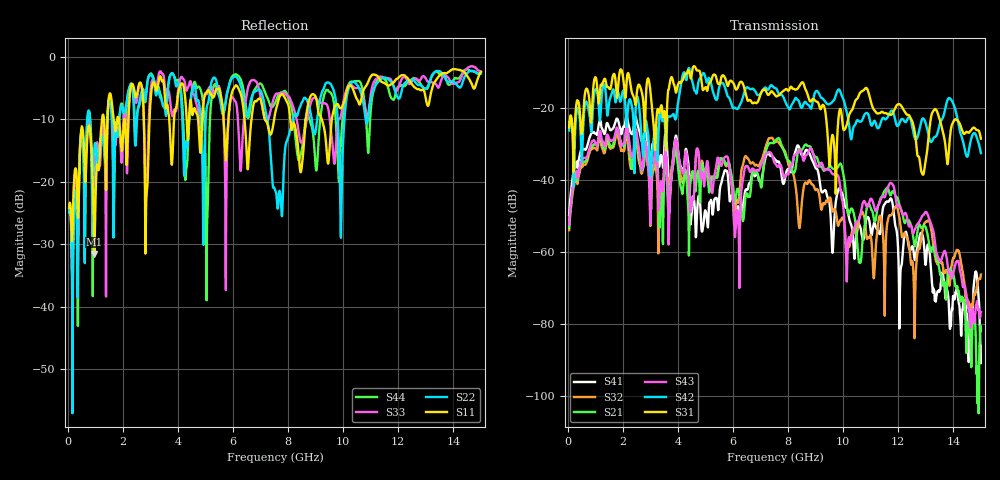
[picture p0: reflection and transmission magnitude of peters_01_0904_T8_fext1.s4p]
# MHZ S RI R 50.00
! FREQ  S11  S12  S13  S14
!  S21  S22  S23  S24
!  S31  S32  S33  S34
!  S41  S42  S43  S44
!  REAL  IMAG  REAL  IMAG  REAL  IMAG  REAL  IMAG
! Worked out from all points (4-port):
!   1496 points, 50 MHz to 15 GHz, reference 50 ohm
!   strongest paths, dB at 50 MHz, 3.79 GHz, 7.53 GHz, 11.27 GHz, 15 GHz:
!     S31: -25.3, -11.5, -16.4, -21.4, -28.4
!     S42: -26.2, -22.0, -14.3, -25.5, -32.4
!     S43: -52.3, -37.5, -35.3, -47.1, -76.5
!     S21: -53.0, -37.3, -29.1, -47.0, -81.7
!     S32: -53.8, -35.6, -29.4, -52.1, -66.2
!     S41: -49.6, -36.9, -34.2, -54.0, -90.7
!   lowest |S11| = -31.6 dB at 960 MHz (marker M1), VSWR 1.05, Z = 47.6 - j1.02 ohm
!   |S11| at or under -10 dB: start of sweep to 1.245 GHz; 8.079 GHz to 8.642 GHz (562.9 MHz wide, 6.73 % of centre); 9.224 GHz to 9.588 GHz (363.7 MHz wide, 3.87 % of centre)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
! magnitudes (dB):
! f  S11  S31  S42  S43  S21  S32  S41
! 50 MHz  -24.1  -25.3  -26.2  -52.3  -53.0  -53.8  -49.6
! 960 MHz  -31.6  -12.2  -16.0  -28.9  -29.9  -30.9  -26.7
! 3.02 GHz  -6.3  -16.7  -38.3  -46.2  -48.1  -44.8  -35.1
! 4.9 GHz  -8.7  -14.9  -10.4  -38.0  -35.6  -35.3  -53.5
! 8.72 GHz  -7.7  -16.4  -19.0  -32.5  -30.5  -40.7  -31.9
! 10.15 GHz  -5.1  -24.0  -21.7  -62.1  -48.1  -59.8  -48.0
! 15 GHz  -2.4  -28.4  -32.4  -76.5  -81.7  -66.2  -90.7
